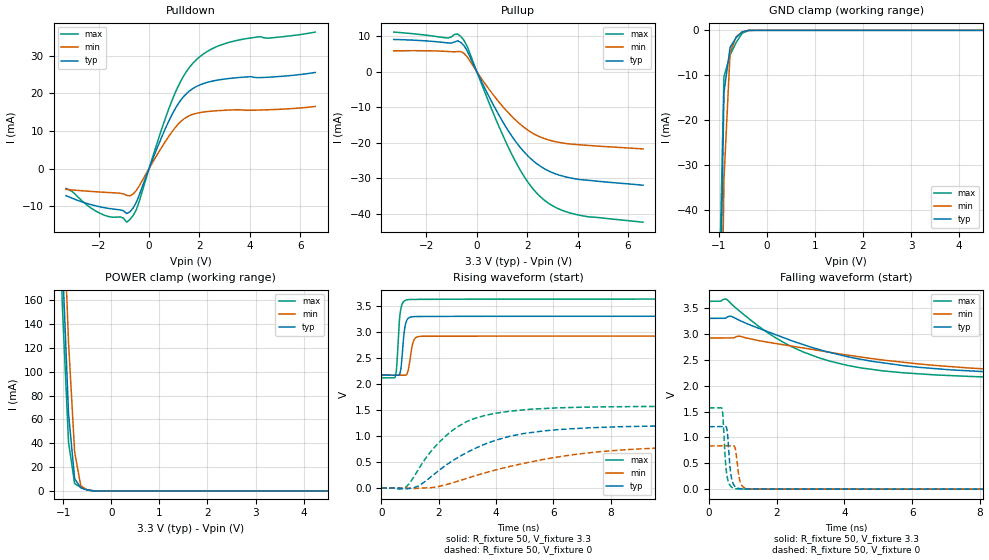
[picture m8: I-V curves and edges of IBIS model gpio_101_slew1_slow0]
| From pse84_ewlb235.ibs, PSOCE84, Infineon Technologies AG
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[Model] gpio_101_slew1_slow0
Model_type I/O
Enable   Active-High
Vinl  =  0.99
Vinh  =  2.31
Vmeas =  1.65
Cref  =  15e-12
| Capacitance   typ   min   max
C_comp   1.09946e-12   1.086232e-12   1.114407e-12
| Variables   typ   min   max
[GND Clamp Reference]   0   0   0
[POWER Clamp Reference]   3.3   2.92   3.63
[Pulldown Reference]   0   0   0
[Pullup Reference]   3.3   2.92   3.63
[Temperature Range]   25   125   -40
[Voltage Range]   3.3   2.92   3.63
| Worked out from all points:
|   slope of the pulldown table from 0 to 0.495 V, typ, clamps not added: 59.8 ohm
|   slope of the pullup table from 0 to 0.495 V, typ, clamps not added: 69.5 ohm
|   GND clamp passes 1 mA (typ) near -0.57 V on its own axis
|   POWER clamp passes 1 mA (typ) near -0.52 V on its own axis
|   falling waveform, R_fixture 50, V_fixture 3.3: 20-80 % time 4.02ns typ, 5.9ns min, 2.8ns max; typ from 3.3 V to 2.17 V
|   falling waveform, R_fixture 50, V_fixture 0: 20-80 % time 96.7ps typ, 105ps min, 93.3ps max; typ from 1.21 V to 0 V
|   rising waveform, R_fixture 50, V_fixture 3.3: 20-80 % time 114ps typ, 135ps min, 103ps max; typ from 2.17 V to 3.3 V
|   rising waveform, R_fixture 50, V_fixture 0: 20-80 % time 2.51ns typ, 4.24ns min, 1.67ns max; typ from 0 V to 1.21 V
[GND Clamp]
| Voltage   I(typ)   I(min)   I(max)
-1.65V    -892.5mA   -911.9mA   -883.9mA
-1.015V   -92.32mA   -129.7mA   -71.28mA
-888.3mV  -13.83mA   -33.21mA   -10.31mA
-761.4mV  -3.792mA   -4.944mA   -5.509mA
-634.5mV  -1.622mA   -1.436mA   -2.707mA
-507.6mV  -326.2uA   -352.3uA   -651.6uA
-380.7mV  -13.48uA   -32.14uA   -19.55uA
-253.8mV  -189.4nA   -1.276uA   -466.7nA
6.6V      0A         0A         0A
[POWER Clamp]
| Voltage   I(typ)   I(min)   I(max)
-1.523V   838.1mA    872.9mA    823.9mA
-1.142V   346.5mA    405.1mA    310.5mA
-1.015V   193mA      257.4mA    153.9mA
-888.3mV  64.97mA    124.9mA    40.96mA
-761.4mV  10.28mA    32.7mA     6.184mA
-634.5mV  2.553mA    4.346mA    3.067mA
-507.6mV  805.9uA    960.7uA    1.159mA
-253.8mV  1.454uA    10.02uA    1.678uA
6.6V      0A         0A         0A
[Pulldown]
| Voltage   I(typ)   I(min)   I(max)
-3.3V     -7.203mA   -5.558mA   -5.309mA
-2.03V    -10.05mA   -6.209mA   -11.63mA
-1.142V   -11mA      -6.584mA   -12.87mA
-888.3mV  -11.97mA   -7.138mA   -14.27mA
-507.6mV  -8.987mA   -5.838mA   -10.98mA
341.4mV   5.791mA    3.893mA    7.243mA
910.3mV   14.34mA    9.777mA    18.1mA
1.366V    19.09mA    13.11mA    24.54mA
1.821V    21.6mA     14.58mA    28.57mA
2.503V    23.23mA    15.27mA    31.85mA
3.3V      24.03mA    15.58mA    33.77mA
6.6V      25.56mA    16.5mA     36.29mA
[Pullup]
| Voltage   I(typ)   I(min)   I(max)
-3.3V     9.072mA    5.875mA    11.15mA
-1.142V   8.101mA    5.689mA    9.493mA
-761.4mV  8.711mA    5.684mA    10.6mA
-634.5mV  8.24mA     5.672mA    9.896mA
-380.7mV  5.841mA    4.169mA    7.086mA
682.8mV   -9.682mA   -6.78mA    -12.13mA
1.479V    -19.03mA   -13.2mA    -24.52mA
2.048V    -23.85mA   -16.55mA   -31.28mA
2.731V    -27.5mA    -18.94mA   -36.43mA
3.3V      -29.17mA   -19.95mA   -38.76mA
4.051V    -30.32mA   -20.54mA   -40.36mA
6.6V      -31.95mA   -21.74mA   -42.36mA
[Ramp]
dV/dt_r   0.724504/2.50945n  0.501631/4.24n  0.941981/1.67009n
dV/dt_f   0.678582/4.01933n  0.451029/5.9036n  0.908165/2.79761n
R_load = 50
[Falling Waveform]
R_fixture = 50
V_fixture = 3.3
V_fixture_min = 2.92
V_fixture_max = 3.63
| Time   V(typ)   V(min)   V(max)
0s        3.3V       2.92V      3.63V
509.7ps   3.313V     2.92V      3.671V
663.5ps   3.339V     2.92V      3.577V
1.493ns   3.103V     2.867V     3.134V
2.456ns   2.865V     2.763V     2.748V
3.566ns   2.643V     2.643V     2.474V
4.497ns   2.508V     2.551V     2.342V
8.434ns   2.26V      2.314V     2.163V
13.9ns    2.188V     2.206V     2.121V
800ns     2.169V     2.168V     2.116V
[Falling Waveform]
R_fixture = 50
V_fixture = 0
V_fixture_min = 0
V_fixture_max = 0
| Time   V(typ)   V(min)   V(max)
0s        1.208V     836.1mV    1.57V
384.5ps   1.208V     835.9mV    1.551V
484.3ps   1.211V     836mV      547.1mV
526.8ps   1.167V     836.1mV    280.3mV
606.6ps   533.5mV    836.1mV    88.96mV
663.1ps   220.9mV    836.3mV    41.53mV
742.9ps   72.07mV    834.1mV    14.43mV
929.9ps   7.411mV    125.6mV    3.571mV
1.219ns   2.191mV    4.565mV    2.663mV
800ns     15.82nV    505.1nV    9.033nV
[Rising Waveform]
R_fixture = 50
V_fixture = 3.3
V_fixture_min = 2.92
V_fixture_max = 3.63
| Time   V(typ)   V(min)   V(max)
0s        2.169V     2.168V     2.116V
495.3ps   2.169V     2.168V     2.149V
541.9ps   2.169V     2.168V     2.352V
648.2ps   2.196V     2.168V     3.304V
779.8ps   2.886V     2.168V     3.582V
900.2ps   3.231V     2.195V     3.616V
1.089ns   3.291V     2.754V     3.623V
1.189ns   3.294V     2.881V     3.624V
2.195ns   3.297V     2.918V     3.628V
800ns     3.3V       2.92V      3.63V
[Rising Waveform]
R_fixture = 50
V_fixture = 0
V_fixture_min = 0
V_fixture_max = 0
| Time   V(typ)   V(min)   V(max)
0s        16.07nV    504.8nV    9.389nV
852.6ps   -17.25mV   -513.6uV   14.64mV
1.306ns   43.68mV    -3.442mV   366mV
2.224ns   425.3mV    58.06mV    986.9mV
2.979ns   679.1mV    184.1mV    1.275V
3.605ns   840.1mV    288.9mV    1.393V
4.5ns     996.3mV    416.3mV    1.477V
6.208ns   1.124V     600.5mV    1.541V
10.88ns   1.198V     789mV      1.569V
800ns     1.208V     836.1mV    1.57V
